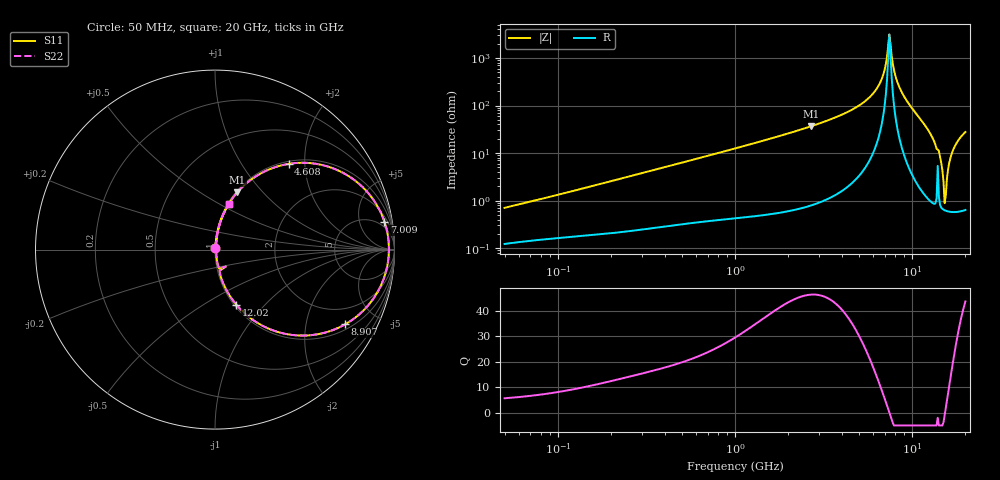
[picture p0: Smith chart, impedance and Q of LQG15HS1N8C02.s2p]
!Murata Part Number: LQG15HS1N8C02
!These Parameters are Measured in Series Mode Connection
!  o--[Z]--o
!Port1  Port2
!  o-------o
!Freq. Start=50[MHz] Stop=20[GHz], 401[Steps]
# Hz S RI R 50
!Freq.(Hz) S11(Real) S11(Imag) S21(Real) S21(Imag) S12(Real) S12(Imag) S22(Real) S22(Imag)
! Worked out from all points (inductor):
!   401 points, 50 MHz to 20 GHz, reference 50 ohm
!   read as one part in series: L = 2.16 nH near 51.52 MHz
!   highest Q = 46.3 at 2.687 GHz (marker M1), where L = 2.17 nH
!   self-resonance near 7.442 GHz
!   S11 on the Smith chart (normalised r, x): 50 MHz: 1.00, +0.01; 4.608 GHz: 1.05, +1.66; 7.009 GHz: 3, +11; 8.907 GHz: 1.21, -3.35; 12.02 GHz: 1.02, -0.70; 20 GHz: 1.01, +0.55
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5e7  0.00127 0.00693  0.9987 -0.00693  0.9987 -0.00693  0.00127 0.00693
1.364002e8  0.00211 0.0176  0.9979 -0.0176  0.9979 -0.0176  0.00211 0.0176
3.721004e8  0.00492 0.0466  0.9951 -0.0466  0.9951 -0.0466  0.00492 0.0466
1e9  0.0194 0.1221  0.9806 -0.1221  0.9806 -0.1221  0.0194 0.1221
2.687447e9  0.1237 0.3186  0.8763 -0.3186  0.8763 -0.3186  0.1237 0.3186
2.728004e9  0.1276 0.3231  0.8724 -0.3231  0.8724 -0.3231  0.1276 0.3231
4.608136e9  0.4105 0.4777  0.5895 -0.4777  0.5895 -0.4777  0.4105 0.4777
6.125241e9  0.7763 0.3877  0.2237 -0.3877  0.2237 -0.3877  0.7763 0.3877
6.601595e9  0.8814 0.2794  0.1186 -0.2794  0.1186 -0.2794  0.8814 0.2794
7.009217e9  0.9442 0.1553  0.0558 -0.1553  0.0558 -0.1553  0.9442 0.1553
7.442007e9  0.9692 0.00311  0.0308 -0.00311  0.0308 -0.00311  0.9692 0.00311
7.668323e9  0.9624 -0.0786  0.0376 0.0786  0.0376 0.0786  0.9624 -0.0786
8.141811e9  0.905 -0.2379  0.095 0.2379  0.095 0.2379  0.905 -0.2379
8.907419e9  0.7254 -0.4165  0.2746 0.4165  0.2746 0.4165  0.7254 -0.4165
1.004137e10  0.4265 -0.4752  0.5735 0.4752  0.5735 0.4752  0.4265 -0.4752
1.201863e10  0.1182 -0.3062  0.8818 0.3062  0.8818 0.3062  0.1182 -0.3062
1.417136e10  0.0234 -0.1063  0.9766 0.1063  0.9766 0.1063  0.0234 -0.1063
1.527346e10  0.00627 -0.00614  0.9937 0.00614  0.9937 0.00614  0.00627 -0.00614
1.573793e10  0.00679 0.0284  0.9932 -0.0284  0.9932 -0.0284  0.00679 0.0284
1.621653e10  0.00962 0.0614  0.9904 -0.0614  0.9904 -0.0614  0.00962 0.0614
1.696185e10  0.0176 0.1083  0.9824 -0.1083  0.9824 -0.1083  0.0176 0.1083
2e10  0.0765 0.2546  0.9235 -0.2546  0.9235 -0.2546  0.0765 0.2546
